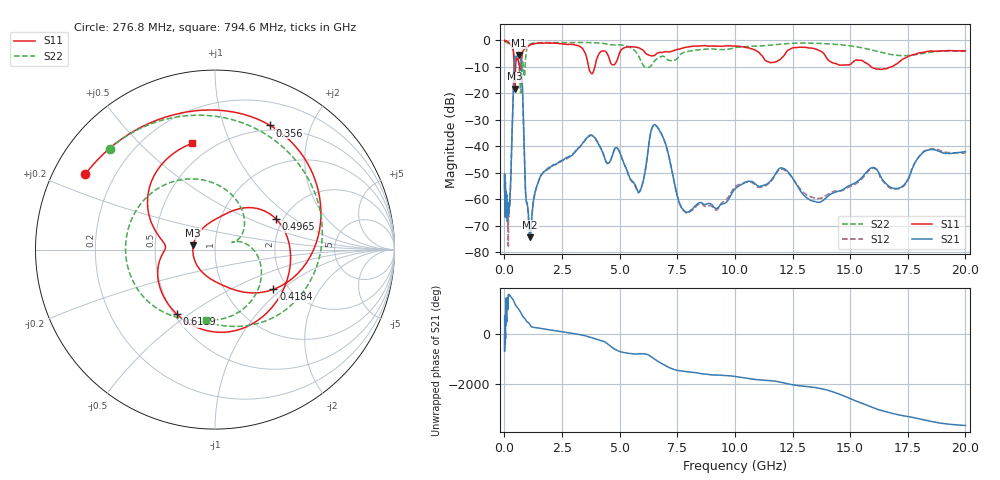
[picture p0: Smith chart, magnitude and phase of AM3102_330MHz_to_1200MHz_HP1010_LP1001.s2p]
! Date/Time: Tue, Sep 11, 2018 5:19 PM
! Network Analyzer: Agilent Technologies E8362B Rev: A.07.50.63
! Sweep from 0.010 to 20.000 GHz, 1601 Points, Sweep Type: LOG
! Power Supply: 4.949 V, 0.001 A
# Hz S DB R 50
!freq MagS11 AngS11 MagS21 AngS21 MagS12 AngS12 MagS22 AngS22
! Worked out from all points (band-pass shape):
!   1601 points, 10 MHz to 20 GHz, reference 50 ohm
!   highest |S21| = -5.45 dB at 635.6 MHz (marker M1); lowest = -74.3 dB at 1.124 GHz (marker M2)
!   |S21| within 3 dB of the highest: 433.8 MHz to 728.4 MHz (294.6 MHz wide, 50.7 % of centre)
!   lowest |S11| = -18.2 dB at 451.5 MHz (marker M3), VSWR 1.28, Z = 39.1 + j1.84 ohm
!   |S11| at or under -10 dB: 424.6 MHz to 482.8 MHz (58.2 MHz wide, 12.8 % of centre); 3.653 GHz to 3.924 GHz (271.8 MHz wide, 7.18 % of centre); 15.91 GHz to 16.77 GHz (855.4 MHz wide, 5.24 % of centre)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
!   |S22| runs from -19.8 to -0.2 dB; largest |S21 - S12| = 0.01
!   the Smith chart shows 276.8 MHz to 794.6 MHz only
!   S11 on the Smith chart (normalised r, x): 276.8 MHz: 0.10, +0.27; 356 MHz: 0.45, +1.44; 418.4 MHz: 1.68, -0.88; 496.5 MHz: 1.84, +0.74; 611.9 MHz: 0.52, -0.45; 794.6 MHz: 0.39, +0.73
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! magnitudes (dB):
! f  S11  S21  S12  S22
! 10 MHz  0.0  -53.7  -56.4  -0.2
! 35.55 MHz  0.0  -63.1  -63.8  -0.4
! 48.18 MHz  0.0  -59.1  -53.6  -0.5
! 126.4 MHz  -0.4  -64.8  -63.5  -0.9
! 168.9 MHz  -0.6  -65.7  -75.8  -1.1
! 276.8 MHz  -1.6  -52.7  -52.7  -1.8
! 356 MHz  -2.4  -28.1  -28.2  -3.4
! 418.4 MHz  -8.1  -10.9  -10.9  -6.2
! 447.2 MHz  -18.0  -7.2  -7.2  -7.7
! 451.5 MHz  -18.2  -6.9  -6.9  -7.7
! 496.5 MHz  -8.4  -6.1  -6.1  -6.4
! 611.9 MHz  -7.6  -5.5  -5.7  -8.1
! 635.6 MHz  -8.6  -5.4  -5.5  -9.9
! 794.6 MHz  -4.4  -20.6  -20.7  -8.1
! 920.7 MHz  -2.9  -57.6  -57.5  -6.8
! 1.124 GHz  -1.7  -74.3  -75.1  -1.3
! 1.59 GHz  -1.0  -50.8  -51.0  -0.8
! 3.775 GHz  -12.5  -35.8  -35.7  -0.8
! 5.652 GHz  -2.5  -54.2  -54.6  -3.8
! 6.58 GHz  -5.2  -32.1  -32.2  -7.2
! 7.958 GHz  -2.4  -64.8  -65.3  -4.1
! 20 GHz  -3.9  -42.0  -42.5  -4.0
